| TEXAS INSTRUMENTS INCORPORATED
| Standard Linear and Logic Group
| IBIS Model of SN74AHCT139
| DUAL 2-LINE TO 4-LINE DECODERS/DEMULTIPLEXERS
| This file contains package information for the following:
|  SOIC 16-pin (D) package as [Component] AHCT139_D
|  SSOP 16-pin (DB) package as [Component] AHCT139_DB
|  TVSOP 16-pin (DGV) package as [Component] AHCT139_DGV
|  PDIP 16-pin (N) package as [Component] AHCT139_N
|  SOP 16-pin (NS) package as [Component] AHCT139_NS
|  TSSOP 16-pin (PW) package as [Component] AHCT139_PW
| This device can be powered at the following Vccs:
|  5 volt Vcc
| This file provides unique models under the [Model Selector] for each Vcc.
| For operation at a specific Vcc, select the appropriate model after each
| [Model Selector] keyword.
[IBIS Ver]   3.2
[Comment char]  |_char
[File Name]   sn74ahct139.ibs
[File Rev]   1.1 | a_die
[Date]   November 20, 2002
[Source]   Data created from TI-SPICE simulations at TI-SLL.
[Notes]   The following is an IBIS list for the AHCT139.
   Please contact sllibis@ti.com with questions and
   comments concerning SLL IBIS models.
   -This IBIS model is created from a BA (back annotated
   netlist).
   -Power clamp data deleted as there is no power-clamp diode.
[Disclaimer] Property of Texas Instruments Incorporated.  Unauthorized
   reproduction and/or distribution is strictly prohibited.
   This product is protected under copyright law.
   Created  2002, (C) Copyright  2002, Texas Instruments
   Incorporated, All Rights Reserved
   UNLESS THERE IS A SIGNED, WRITTEN AGREEMENT TO THE
   CONTRARY, TEXAS INSTRUMENTS (TI) IS PROVIDING THE IBIS
   MODELS  AND WITHOUT ANY WARRANTY, EXPRESSED OR
   IMPLIED.  TI assumes no liability for:
   1) the accuracy of the IBIS models provided to your
   company;
   2) the proper functioning of these IBIS Models in your
   design or for any resulting applications; or
   3) infringement of patents, copyrights or intellectual
   property rights resulting from your use of these IBIS
   models.
   TI provides IBIS Models as a service to our customers.
   You and your company shall not distribute, sell or give
   these models to anyone else without prior written
   permission from TI.
   TI reserves the right to make changes to our products or
   to discontinue any semiconductor product or service
   without notice, and advises our customers to obtain the
   latest version of relevant information to verify, before
   placing orders, that the information being relied on is
   current.
   Please be aware that your receipt and use of the IBIS
   information provided shall serve as acceptance of these
   terms and conditions.  If you do not accept these terms,
   you should return or destroy the IBIS models and any
   other accompanying information immediately.
| Component AHCT139_D 16-pin SOIC
[Component]   AHCT139_D
[Manufacturer]   Texas Instruments, Inc.
[Package]
|   typ   min   max
R_pkg   3.900e-02   2.800e-02   4.900e-02
L_pkg   3.453e-09   2.350e-09   4.375e-09
C_pkg   5.210e-13   2.540e-13   7.080e-13
[Pin]   signal_name   model_name   R_pin   L_pin   C_pin
1   1NG   AHCT139_ENABLE   4.200e-02   4.336e-09   7.030e-13
2   1A   AHCT139_SELECT   4.900e-02   3.778e-09   6.340e-13
3   1B   AHCT139_SELECT   2.800e-02   3.449e-09   5.180e-13
4   1Y0   AHCT139_OUT   2.900e-02   2.393e-09   2.540e-13
5   1Y1   AHCT139_OUT   2.800e-02   2.350e-09   2.640e-13
6   1Y2   AHCT139_OUT   4.800e-02   3.312e-09   4.830e-13
7   1Y3   AHCT139_OUT   4.300e-02   3.629e-09   6.040e-13
8   GND   GND   4.400e-02   4.375e-09   7.080e-13
9   2Y3   AHCT139_OUT   4.200e-02   4.336e-09   7.030e-13
10   2Y2   AHCT139_OUT   4.900e-02   3.778e-09   6.340e-13
11   2Y1   AHCT139_OUT   2.800e-02   3.449e-09   5.180e-13
12   2Y0   AHCT139_OUT   2.900e-02   2.393e-09   2.550e-13
13   2B   AHCT139_SELECT   2.800e-02   2.350e-09   2.640e-13
14   2A   AHCT139_SELECT   4.800e-02   3.312e-09   4.830e-13
15   2NG   AHCT139_ENABLE   4.300e-02   3.629e-09   6.040e-13
16   VCC   POWER   4.400e-02   4.375e-09   7.080e-13
| Component AHCT139_DB 16-pin SSOP
[Component]   AHCT139_DB
[Manufacturer]   Texas Instruments, Inc.
[Package]
|   typ   min   max
R_pkg   4.800e-02   4.600e-02   5.000e-02
L_pkg   3.536e-09   3.213e-09   3.798e-09
C_pkg   3.760e-13   3.140e-13   4.400e-13
[Pin]   signal_name   model_name   R_pin   L_pin   C_pin
1   1NG   AHCT139_ENABLE   4.800e-02   3.797e-09   3.770e-13
2   1A   AHCT139_SELECT   4.600e-02   3.723e-09   4.400e-13
3   1B   AHCT139_SELECT   4.800e-02   3.409e-09   3.720e-13
4   1Y0   AHCT139_OUT   4.900e-02   3.213e-09   3.140e-13
5   1Y1   AHCT139_OUT   4.900e-02   3.213e-09   3.140e-13
6   1Y2   AHCT139_OUT   4.800e-02   3.409e-09   3.720e-13
7   1Y3   AHCT139_OUT   4.600e-02   3.723e-09   4.400e-13
8   GND   GND   4.800e-02   3.798e-09   3.770e-13
9   2Y3   AHCT139_OUT   4.800e-02   3.797e-09   3.770e-13
10   2Y2   AHCT139_OUT   4.600e-02   3.725e-09   4.400e-13
11   2Y1   AHCT139_OUT   4.800e-02   3.409e-09   3.720e-13
12   2Y0   AHCT139_OUT   4.900e-02   3.214e-09   3.140e-13
13   2B   AHCT139_SELECT   5.000e-02   3.216e-09   3.140e-13
14   2A   AHCT139_SELECT   4.800e-02   3.409e-09   3.720e-13
15   2NG   AHCT139_ENABLE   4.700e-02   3.729e-09   4.400e-13
16   VCC   POWER   4.800e-02   3.797e-09   3.770e-13
| Component AHCT139_DGV 16-pin TVSOP
[Component]   AHCT139_DGV
[Manufacturer]   Texas Instruments, Inc.
[Package]
|   typ   min   max
R_pkg   3.900e-02   3.300e-02   4.500e-02
L_pkg   2.543e-09   2.320e-09   2.938e-09
C_pkg   3.860e-13   3.340e-13   4.490e-13
[Pin]   signal_name   model_name   R_pin   L_pin   C_pin
1   1NG   AHCT139_ENABLE   3.500e-02   2.907e-09   4.170e-13
2   1A   AHCT139_SELECT   4.200e-02   2.558e-09   4.460e-13
3   1B   AHCT139_SELECT   3.800e-02   2.341e-09   3.450e-13
4   1Y0   AHCT139_OUT   3.800e-02   2.320e-09   3.340e-13
5   1Y1   AHCT139_OUT   3.900e-02   2.322e-09   3.340e-13
6   1Y2   AHCT139_OUT   3.800e-02   2.353e-09   3.420e-13
7   1Y3   AHCT139_OUT   4.000e-02   2.536e-09   4.410e-13
8   GND   GND   3.300e-02   2.897e-09   4.180e-13
9   2Y3   AHCT139_OUT   3.500e-02   2.927e-09   4.190e-13
10   2Y2   AHCT139_OUT   4.500e-02   2.632e-09   4.490e-13
11   2Y1   AHCT139_OUT   3.900e-02   2.368e-09   3.470e-13
12   2Y0   AHCT139_OUT   3.900e-02   2.330e-09   3.350e-13
13   2B   AHCT139_SELECT   3.900e-02   2.320e-09   3.350e-13
14   2A   AHCT139_SELECT   3.900e-02   2.361e-09   3.450e-13
15   2NG   AHCT139_ENABLE   4.100e-02   2.573e-09   4.460e-13
16   VCC   POWER   3.500e-02   2.938e-09   4.200e-13
| Component AHCT139_N 16-pin PDIP
[Component]   AHCT139_N
[Manufacturer]   Texas Instruments, Inc.
[Package]
|   typ   min   max
R_pkg   5.600e-02   5.200e-02   6.300e-02
L_pkg   7.637e-09   5.451e-09   1.053e-08
C_pkg   5.280e-13   3.350e-13   8.930e-13
[Pin]   signal_name   model_name   R_pin   L_pin   C_pin
1   1NG   AHCT139_ENABLE   5.800e-02   1.053e-08   8.920e-13
2   1A   AHCT139_SELECT   6.200e-02   8.759e-09   5.350e-13
3   1B   AHCT139_SELECT   5.200e-02   7.146e-09   3.870e-13
4   1Y0   AHCT139_OUT   5.300e-02   5.451e-09   4.080e-13
5   1Y1   AHCT139_OUT   5.300e-02   5.513e-09   3.700e-13
6   1Y2   AHCT139_OUT   5.300e-02   6.304e-09   3.360e-13
7   1Y3   AHCT139_OUT   5.700e-02   7.830e-09   5.030e-13
8   GND   GND   5.600e-02   9.581e-09   8.050e-13
9   2Y3   AHCT139_OUT   5.800e-02   9.603e-09   8.070e-13
10   2Y2   AHCT139_OUT   6.200e-02   7.864e-09   5.030e-13
11   2Y1   AHCT139_OUT   5.200e-02   6.295e-09   3.350e-13
12   2Y0   AHCT139_OUT   5.300e-02   5.499e-09   3.560e-13
13   2B   AHCT139_SELECT   5.300e-02   5.452e-09   4.040e-13
14   2A   AHCT139_SELECT   5.300e-02   7.156e-09   3.870e-13
15   2NG   AHCT139_ENABLE   6.300e-02   8.740e-09   5.340e-13
16   VCC   POWER   5.600e-02   1.048e-08   8.930e-13
| Component AHCT139_NS 16-pin SOP
[Component]   AHCT139_NS
[Manufacturer]   Texas Instruments, Inc.
[Package]
|   typ   min   max
R_pkg   4.200e-02   3.500e-02   4.900e-02
L_pkg   3.147e-09   2.164e-09   4.219e-09
C_pkg   4.040e-13   2.410e-13   5.620e-13
[Pin]   signal_name   model_name   R_pin   L_pin   C_pin
1   1NG   AHCT139_ENABLE   4.900e-02   4.215e-09   5.620e-13
2   1A   AHCT139_SELECT   4.600e-02   3.675e-09   4.800e-13
3   1B   AHCT139_SELECT   3.700e-02   2.527e-09   3.320e-13
4   1Y0   AHCT139_OUT   3.500e-02   2.164e-09   2.410e-13
5   1Y1   AHCT139_OUT   3.500e-02   2.164e-09   2.410e-13
6   1Y2   AHCT139_OUT   3.700e-02   2.527e-09   3.320e-13
7   1Y3   AHCT139_OUT   4.600e-02   3.675e-09   4.800e-13
8   GND   GND   4.900e-02   4.215e-09   5.620e-13
9   2Y3   AHCT139_OUT   4.900e-02   4.219e-09   5.620e-13
10   2Y2   AHCT139_OUT   4.600e-02   3.679e-09   4.800e-13
11   2Y1   AHCT139_OUT   3.700e-02   2.531e-09   3.330e-13
12   2Y0   AHCT139_OUT   3.500e-02   2.168e-09   2.410e-13
13   2B   AHCT139_SELECT   3.500e-02   2.168e-09   2.410e-13
14   2A   AHCT139_SELECT   3.700e-02   2.531e-09   3.330e-13
15   2NG   AHCT139_ENABLE   4.600e-02   3.679e-09   4.800e-13
16   VCC   POWER   4.900e-02   4.219e-09   5.620e-13
| Component AHCT139_PW 16-pin TSSOP
[Component]   AHCT139_PW
[Manufacturer]   Texas Instruments, Inc.
[Package]
|   typ   min   max
R_pkg   4.500e-02   3.800e-02   5.100e-02
L_pkg   2.593e-09   2.447e-09   3.080e-09
C_pkg   2.810e-13   2.430e-13   3.770e-13
[Pin]   signal_name   model_name   R_pin   L_pin   C_pin
1   1NG   AHCT139_ENABLE   4.000e-02   3.080e-09   3.770e-13
2   1A   AHCT139_SELECT   3.800e-02   2.458e-09   2.810e-13
3   1B   AHCT139_SELECT   5.100e-02   2.512e-09   2.550e-13
4   1Y0   AHCT139_OUT   5.100e-02   2.447e-09   2.430e-13
5   1Y1   AHCT139_OUT   5.100e-02   2.447e-09   2.430e-13
6   1Y2   AHCT139_OUT   5.100e-02   2.512e-09   2.550e-13
7   1Y3   AHCT139_OUT   3.800e-02   2.458e-09   2.810e-13
8   GND   GND   4.000e-02   3.080e-09   3.770e-13
9   2Y3   AHCT139_OUT   3.900e-02   2.832e-09   3.160e-13
10   2Y2   AHCT139_OUT   3.800e-02   2.460e-09   2.790e-13
11   2Y1   AHCT139_OUT   5.100e-02   2.512e-09   2.550e-13
12   2Y0   AHCT139_OUT   5.100e-02   2.447e-09   2.430e-13
13   2B   AHCT139_SELECT   5.100e-02   2.447e-09   2.430e-13
14   2A   AHCT139_SELECT   5.100e-02   2.512e-09   2.550e-13
15   2NG   AHCT139_ENABLE   3.800e-02   2.459e-09   2.790e-13
16   VCC   POWER   3.900e-02   2.832e-09   3.160e-13
| Models and submodels in the file (3): AHCT139_ENABLE (Input), AHCT139_SELECT (Input), AHCT139_OUT (Output)
